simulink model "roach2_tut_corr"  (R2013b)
settings: Solver=VariableStepDiscrete  SolverMode=SingleTasking  StartTime=0.0  StopTime=100  RelTol=1e-3
undefined symbols (not defined in the file): add_latency, addr_width, Bit, bitfield, BitWidth, bram_latency, burst_size, casper_library_scopes, conv_latency, data_width, DelayLen, fan_latency, FFTSize, FFTStage, getfield, increment, led, Location, Lower, mult_latency, mux_latency, n_bits, n_bits_data, n_inputs, n_streams, n_taps, neg_latency, negate_latency, nsamples, pfb_size, pulse_len, reset_period, ROACH, ROACH2, snapshot, sx475t, sync_period, sync_period_bits, Upper, UseCounter, Width
libraries: xbsIndex_r4 x24444, casper_library_misc x73, xbsReplacements_r4 x34, casper_library_delays x14, xps_library x7
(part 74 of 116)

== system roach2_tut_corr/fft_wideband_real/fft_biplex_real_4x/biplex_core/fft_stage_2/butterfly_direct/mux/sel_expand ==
  bus_in : Inport
  reinterpret{1..16} (16 alike) : xbsIndex_r4/Reinterpret  force_arith_type=on  arith_type=Unsigned  force_bin_pt=on  bin_pt=0  block_type=reinterpret
  slice1 : xbsIndex_r4/Slice  nbits=1  boolean_output=off  mode=Upper Bit Location + Width  bit1=-15  base1=MSB of Input  bit0=0  base0=LSB of Input  dbl_ovrd=off  block_type=slice
  slice10 : xbsIndex_r4/Slice  nbits=1  boolean_output=off  mode=Upper Bit Location + Width  bit1=-6  base1=MSB of Input  bit0=0  base0=LSB of Input  dbl_ovrd=off  block_type=slice
  slice11 : xbsIndex_r4/Slice  nbits=1  boolean_output=off  mode=Upper Bit Location + Width  bit1=-5  base1=MSB of Input  bit0=0  base0=LSB of Input  dbl_ovrd=off  block_type=slice
  slice12 : xbsIndex_r4/Slice  nbits=1  boolean_output=off  mode=Upper Bit Location + Width  bit1=-4  base1=MSB of Input  bit0=0  base0=LSB of Input  dbl_ovrd=off  block_type=slice
  slice13 : xbsIndex_r4/Slice  nbits=1  boolean_output=off  mode=Upper Bit Location + Width  bit1=-3  base1=MSB of Input  bit0=0  base0=LSB of Input  dbl_ovrd=off  block_type=slice
  slice14 : xbsIndex_r4/Slice  nbits=1  boolean_output=off  mode=Upper Bit Location + Width  bit1=-2  base1=MSB of Input  bit0=0  base0=LSB of Input  dbl_ovrd=off  block_type=slice
  slice15 : xbsIndex_r4/Slice  nbits=1  boolean_output=off  mode=Upper Bit Location + Width  bit1=-1  base1=MSB of Input  bit0=0  base0=LSB of Input  dbl_ovrd=off  block_type=slice
  slice16 : xbsIndex_r4/Slice  nbits=1  boolean_output=off  mode=Upper Bit Location + Width  bit1=0  base1=MSB of Input  bit0=0  base0=LSB of Input  dbl_ovrd=off  block_type=slice
  slice2 : xbsIndex_r4/Slice  nbits=1  boolean_output=off  mode=Upper Bit Location + Width  bit1=-14  base1=MSB of Input  bit0=0  base0=LSB of Input  dbl_ovrd=off  block_type=slice
  slice3 : xbsIndex_r4/Slice  nbits=1  boolean_output=off  mode=Upper Bit Location + Width  bit1=-13  base1=MSB of Input  bit0=0  base0=LSB of Input  dbl_ovrd=off  block_type=slice
  slice4 : xbsIndex_r4/Slice  nbits=1  boolean_output=off  mode=Upper Bit Location + Width  bit1=-12  base1=MSB of Input  bit0=0  base0=LSB of Input  dbl_ovrd=off  block_type=slice
  slice5 : xbsIndex_r4/Slice  nbits=1  boolean_output=off  mode=Upper Bit Location + Width  bit1=-11  base1=MSB of Input  bit0=0  base0=LSB of Input  dbl_ovrd=off  block_type=slice
  slice6 : xbsIndex_r4/Slice  nbits=1  boolean_output=off  mode=Upper Bit Location + Width  bit1=-10  base1=MSB of Input  bit0=0  base0=LSB of Input  dbl_ovrd=off  block_type=slice
  slice7 : xbsIndex_r4/Slice  nbits=1  boolean_output=off  mode=Upper Bit Location + Width  bit1=-9  base1=MSB of Input  bit0=0  base0=LSB of Input  dbl_ovrd=off  block_type=slice
  slice8 : xbsIndex_r4/Slice  nbits=1  boolean_output=off  mode=Upper Bit Location + Width  bit1=-8  base1=MSB of Input  bit0=0  base0=LSB of Input  dbl_ovrd=off  block_type=slice
  slice9 : xbsIndex_r4/Slice  nbits=1  boolean_output=off  mode=Upper Bit Location + Width  bit1=-7  base1=MSB of Input  bit0=0  base0=LSB of Input  dbl_ovrd=off  block_type=slice
  msb_out16 : Outport
  out15 : Outport  Port=2
  out14 : Outport  Port=3
  out13 : Outport  Port=4
  out12 : Outport  Port=5
  out11 : Outport  Port=6
  out10 : Outport  Port=7
  out9 : Outport  Port=8
  out8 : Outport  Port=9
  out7 : Outport  Port=10
  out6 : Outport  Port=11
  out5 : Outport  Port=12
  out4 : Outport  Port=13
  out3 : Outport  Port=14
  out2 : Outport  Port=15
  lsb_out1 : Outport  Port=16
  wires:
  bus_in/1 -> slice16/1, slice15/1, slice14/1, slice13/1, slice12/1, slice11/1, slice10/1, slice9/1, slice8/1, slice7/1, slice6/1, slice5/1, slice4/1, slice3/1, slice2/1, slice1/1
  slice16/1 -> reinterpret16/1
  reinterpret16/1 -> msb_out16/1
  slice15/1 -> reinterpret15/1
  reinterpret15/1 -> out15/1
  slice14/1 -> reinterpret14/1
  reinterpret14/1 -> out14/1
  slice13/1 -> reinterpret13/1
  reinterpret13/1 -> out13/1
  slice12/1 -> reinterpret12/1
  reinterpret12/1 -> out12/1
  slice11/1 -> reinterpret11/1
  reinterpret11/1 -> out11/1
  slice10/1 -> reinterpret10/1
  reinterpret10/1 -> out10/1
  slice9/1 -> reinterpret9/1
  reinterpret9/1 -> out9/1
  slice8/1 -> reinterpret8/1
  reinterpret8/1 -> out8/1
  slice7/1 -> reinterpret7/1
  reinterpret7/1 -> out7/1
  slice6/1 -> reinterpret6/1
  reinterpret6/1 -> out6/1
  slice5/1 -> reinterpret5/1
  reinterpret5/1 -> out5/1
  slice4/1 -> reinterpret4/1
  reinterpret4/1 -> out4/1
  slice3/1 -> reinterpret3/1
  reinterpret3/1 -> out3/1
  slice2/1 -> reinterpret2/1
  reinterpret2/1 -> out2/1
  slice1/1 -> reinterpret1/1
  reinterpret1/1 -> lsb_out1/1

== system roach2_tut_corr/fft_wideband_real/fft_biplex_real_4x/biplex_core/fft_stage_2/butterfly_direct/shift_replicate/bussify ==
  in1 : Inport
  in2 : Inport  Port=2
  in3 : Inport  Port=3
  in4 : Inport  Port=4
  in5 : Inport  Port=5
  in6 : Inport  Port=6
  in7 : Inport  Port=7
  in8 : Inport  Port=8
  in9 : Inport  Port=9
  in10 : Inport  Port=10
  in11 : Inport  Port=11
  in12 : Inport  Port=12
  in13 : Inport  Port=13
  in14 : Inport  Port=14
  in15 : Inport  Port=15
  in16 : Inport  Port=16
  concatenate : xbsIndex_r4/Concat  num_inputs=16  dbl_ovrd=off  block_type=concat
  reinterpret{1..16} (16 alike) : xbsIndex_r4/Reinterpret  force_arith_type=on  arith_type=Unsigned  force_bin_pt=on  bin_pt=0  block_type=reinterpret
  bus_out : Outport
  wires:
  concatenate/1 -> bus_out/1
  in1/1 -> reinterpret1/1
  reinterpret1/1 -> concatenate/1
  in2/1 -> reinterpret2/1
  reinterpret2/1 -> concatenate/2
  in3/1 -> reinterpret3/1
  reinterpret3/1 -> concatenate/3
  in4/1 -> reinterpret4/1
  reinterpret4/1 -> concatenate/4
  in5/1 -> reinterpret5/1
  reinterpret5/1 -> concatenate/5
  in6/1 -> reinterpret6/1
  reinterpret6/1 -> concatenate/6
  in7/1 -> reinterpret7/1
  reinterpret7/1 -> concatenate/7
  in8/1 -> reinterpret8/1
  reinterpret8/1 -> concatenate/8
  in9/1 -> reinterpret9/1
  reinterpret9/1 -> concatenate/9
  in10/1 -> reinterpret10/1
  reinterpret10/1 -> concatenate/10
  in11/1 -> reinterpret11/1
  reinterpret11/1 -> concatenate/11
  in12/1 -> reinterpret12/1
  reinterpret12/1 -> concatenate/12
  in13/1 -> reinterpret13/1
  reinterpret13/1 -> concatenate/13
  in14/1 -> reinterpret14/1
  reinterpret14/1 -> concatenate/14
  in15/1 -> reinterpret15/1
  reinterpret15/1 -> concatenate/15
  in16/1 -> reinterpret16/1
  reinterpret16/1 -> concatenate/16

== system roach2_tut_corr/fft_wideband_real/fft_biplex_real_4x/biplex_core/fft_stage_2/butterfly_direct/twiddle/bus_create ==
  in1 : Inport
  in2 : Inport  Port=2
  concatenate : xbsIndex_r4/Concat  num_inputs=2  dbl_ovrd=off  block_type=concat
  reinterpret1 : xbsIndex_r4/Reinterpret  force_arith_type=on  arith_type=Unsigned  force_bin_pt=on  bin_pt=0  block_type=reinterpret
  reinterpret2 : xbsIndex_r4/Reinterpret  force_arith_type=on  arith_type=Unsigned  force_bin_pt=on  bin_pt=0  block_type=reinterpret
  bus_out : Outport
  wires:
  concatenate/1 -> bus_out/1
  in1/1 -> reinterpret1/1
  reinterpret1/1 -> concatenate/1
  in2/1 -> reinterpret2/1
  reinterpret2/1 -> concatenate/2

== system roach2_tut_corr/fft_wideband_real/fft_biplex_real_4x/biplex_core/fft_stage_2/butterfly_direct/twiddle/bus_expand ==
  bus_in : Inport
  reinterpret1 : xbsIndex_r4/Reinterpret  force_arith_type=on  arith_type=Unsigned  force_bin_pt=on  bin_pt=0  block_type=reinterpret
  reinterpret2 : xbsIndex_r4/Reinterpret  force_arith_type=on  arith_type=Unsigned  force_bin_pt=on  bin_pt=0  block_type=reinterpret
  slice1 : xbsIndex_r4/Slice  nbits=72  boolean_output=off  mode=Upper Bit Location + Width  bit1=-72  base1=MSB of Input  bit0=0  base0=LSB of Input  dbl_ovrd=off  block_type=slice
  slice2 : xbsIndex_r4/Slice  nbits=72  boolean_output=off  mode=Upper Bit Location + Width  bit1=0  base1=MSB of Input  bit0=0  base0=LSB of Input  dbl_ovrd=off  block_type=slice
  msb_out2 : Outport
  lsb_out1 : Outport  Port=2
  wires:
  bus_in/1 -> slice2/1, slice1/1
  slice2/1 -> reinterpret2/1
  reinterpret2/1 -> msb_out2/1
  slice1/1 -> reinterpret1/1
  reinterpret1/1 -> lsb_out1/1

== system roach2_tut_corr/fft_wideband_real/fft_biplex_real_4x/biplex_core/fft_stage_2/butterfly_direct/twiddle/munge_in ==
  din : Inport
  join : Subsystem  AncestorBlock=casper_library_flow_control/bus_create
  reinterpret : xbsIndex_r4/Reinterpret  force_arith_type=on  arith_type=Unsigned  force_bin_pt=on  bin_pt=0  block_type=reinterpret
  reinterpret_out : xbsIndex_r4/Reinterpret  force_arith_type=on  arith_type=Unsigned  force_bin_pt=on  bin_pt=0  block_type=reinterpret
  split : Subsystem  AncestorBlock=casper_library_flow_control/bus_expand
  dout : Outport
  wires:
  reinterpret_out/1 -> dout/1
  din/1 -> reinterpret/1
  reinterpret/1 -> split/1(bus_in)
  join/1(bus_out) -> reinterpret_out/1
  split/1(msb_out8) -> join/1(in1)
  split/3(out6) -> join/2(in2)
  split/5(out4) -> join/3(in3)
  split/7(out2) -> join/4(in4)
  split/2(out7) -> join/5(in5)
  split/4(out5) -> join/6(in6)
  split/6(out3) -> join/7(in7)
  split/8(lsb_out1) -> join/8(in8)

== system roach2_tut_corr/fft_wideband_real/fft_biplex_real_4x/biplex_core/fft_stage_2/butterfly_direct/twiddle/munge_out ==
  din : Inport
  join : Subsystem  AncestorBlock=casper_library_flow_control/bus_create
  reinterpret : xbsIndex_r4/Reinterpret  force_arith_type=on  arith_type=Unsigned  force_bin_pt=on  bin_pt=0  block_type=reinterpret
  reinterpret_out : xbsIndex_r4/Reinterpret  force_arith_type=on  arith_type=Unsigned  force_bin_pt=on  bin_pt=0  block_type=reinterpret
  split : Subsystem  AncestorBlock=casper_library_flow_control/bus_expand
  dout : Outport
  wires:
  reinterpret_out/1 -> dout/1
  din/1 -> reinterpret/1
  reinterpret/1 -> split/1(bus_in)
  join/1(bus_out) -> reinterpret_out/1
  split/1(msb_out8) -> join/1(in1)
  split/5(out4) -> join/2(in2)
  split/2(out7) -> join/3(in3)
  split/6(out3) -> join/4(in4)
  split/3(out6) -> join/5(in5)
  split/7(out2) -> join/6(in6)
  split/4(out5) -> join/7(in7)
  split/8(lsb_out1) -> join/8(in8)

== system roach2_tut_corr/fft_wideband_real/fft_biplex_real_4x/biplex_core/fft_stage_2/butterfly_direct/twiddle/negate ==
  din : Inport
  bussify : Subsystem  AncestorBlock=casper_library_flow_control/bus_create
  debus : Subsystem  AncestorBlock=casper_library_flow_control/bus_expand
  neg{1..4} (4 alike) : xbsIndex_r4/Negate  precision=User Defined  arith_type="Signed  (2's comp)"  n_bits=18  bin_pt=17  quantization=Truncate  overflow=Saturate  en=off  latency=latency  dbl_ovrd=off  block_type=negate
  dout : Outport
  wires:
  din/1 -> debus/1(bus_in)
  debus/1(msb_out4) -> neg1/1
  debus/2(out3) -> neg2/1
  debus/3(out2) -> neg3/1
  debus/4(lsb_out1) -> neg4/1
  neg1/1 -> bussify/1(in1)
  neg2/1 -> bussify/2(in2)
  neg3/1 -> bussify/3(in3)
  neg4/1 -> bussify/4(in4)
  bussify/1(bus_out) -> dout/1

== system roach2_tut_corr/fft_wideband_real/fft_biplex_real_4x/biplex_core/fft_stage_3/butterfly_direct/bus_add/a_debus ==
  bus_in : Inport
  reinterpret{1..8} (8 alike) : xbsIndex_r4/Reinterpret  force_arith_type=on  arith_type="Signed  (2's comp)"  force_bin_pt=on  bin_pt=17  block_type=reinterpret
  slice1 : xbsIndex_r4/Slice  nbits=18  boolean_output=off  mode=Upper Bit Location + Width  bit1=-126  base1=MSB of Input  bit0=0  base0=LSB of Input  dbl_ovrd=off  block_type=slice
  slice2 : xbsIndex_r4/Slice  nbits=18  boolean_output=off  mode=Upper Bit Location + Width  bit1=-108  base1=MSB of Input  bit0=0  base0=LSB of Input  dbl_ovrd=off  block_type=slice
  slice3 : xbsIndex_r4/Slice  nbits=18  boolean_output=off  mode=Upper Bit Location + Width  bit1=-90  base1=MSB of Input  bit0=0  base0=LSB of Input  dbl_ovrd=off  block_type=slice
  slice4 : xbsIndex_r4/Slice  nbits=18  boolean_output=off  mode=Upper Bit Location + Width  bit1=-72  base1=MSB of Input  bit0=0  base0=LSB of Input  dbl_ovrd=off  block_type=slice
  slice5 : xbsIndex_r4/Slice  nbits=18  boolean_output=off  mode=Upper Bit Location + Width  bit1=-54  base1=MSB of Input  bit0=0  base0=LSB of Input  dbl_ovrd=off  block_type=slice
  slice6 : xbsIndex_r4/Slice  nbits=18  boolean_output=off  mode=Upper Bit Location + Width  bit1=-36  base1=MSB of Input  bit0=0  base0=LSB of Input  dbl_ovrd=off  block_type=slice
  slice7 : xbsIndex_r4/Slice  nbits=18  boolean_output=off  mode=Upper Bit Location + Width  bit1=-18  base1=MSB of Input  bit0=0  base0=LSB of Input  dbl_ovrd=off  block_type=slice
  slice8 : xbsIndex_r4/Slice  nbits=18  boolean_output=off  mode=Upper Bit Location + Width  bit1=0  base1=MSB of Input  bit0=0  base0=LSB of Input  dbl_ovrd=off  block_type=slice
  msb_out8 : Outport
  out7 : Outport  Port=2
  out6 : Outport  Port=3
  out5 : Outport  Port=4
  out4 : Outport  Port=5
  out3 : Outport  Port=6
  out2 : Outport  Port=7
  lsb_out1 : Outport  Port=8
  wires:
  bus_in/1 -> slice8/1, slice7/1, slice6/1, slice5/1, slice4/1, slice3/1, slice2/1, slice1/1
  slice8/1 -> reinterpret8/1
  reinterpret8/1 -> msb_out8/1
  slice7/1 -> reinterpret7/1
  reinterpret7/1 -> out7/1
  slice6/1 -> reinterpret6/1
  reinterpret6/1 -> out6/1
  slice5/1 -> reinterpret5/1
  reinterpret5/1 -> out5/1
  slice4/1 -> reinterpret4/1
  reinterpret4/1 -> out4/1
  slice3/1 -> reinterpret3/1
  reinterpret3/1 -> out3/1
  slice2/1 -> reinterpret2/1
  reinterpret2/1 -> out2/1
  slice1/1 -> reinterpret1/1
  reinterpret1/1 -> lsb_out1/1

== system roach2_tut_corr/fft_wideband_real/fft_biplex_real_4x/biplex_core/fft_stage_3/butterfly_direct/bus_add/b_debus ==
  bus_in : Inport
  reinterpret{1..8} (8 alike) : xbsIndex_r4/Reinterpret  force_arith_type=on  arith_type="Signed  (2's comp)"  force_bin_pt=on  bin_pt=17  block_type=reinterpret
  slice1 : xbsIndex_r4/Slice  nbits=19  boolean_output=off  mode=Upper Bit Location + Width  bit1=-133  base1=MSB of Input  bit0=0  base0=LSB of Input  dbl_ovrd=off  block_type=slice
  slice2 : xbsIndex_r4/Slice  nbits=19  boolean_output=off  mode=Upper Bit Location + Width  bit1=-114  base1=MSB of Input  bit0=0  base0=LSB of Input  dbl_ovrd=off  block_type=slice
  slice3 : xbsIndex_r4/Slice  nbits=19  boolean_output=off  mode=Upper Bit Location + Width  bit1=-95  base1=MSB of Input  bit0=0  base0=LSB of Input  dbl_ovrd=off  block_type=slice
  slice4 : xbsIndex_r4/Slice  nbits=19  boolean_output=off  mode=Upper Bit Location + Width  bit1=-76  base1=MSB of Input  bit0=0  base0=LSB of Input  dbl_ovrd=off  block_type=slice
  slice5 : xbsIndex_r4/Slice  nbits=19  boolean_output=off  mode=Upper Bit Location + Width  bit1=-57  base1=MSB of Input  bit0=0  base0=LSB of Input  dbl_ovrd=off  block_type=slice
  slice6 : xbsIndex_r4/Slice  nbits=19  boolean_output=off  mode=Upper Bit Location + Width  bit1=-38  base1=MSB of Input  bit0=0  base0=LSB of Input  dbl_ovrd=off  block_type=slice
  slice7 : xbsIndex_r4/Slice  nbits=19  boolean_output=off  mode=Upper Bit Location + Width  bit1=-19  base1=MSB of Input  bit0=0  base0=LSB of Input  dbl_ovrd=off  block_type=slice
  slice8 : xbsIndex_r4/Slice  nbits=19  boolean_output=off  mode=Upper Bit Location + Width  bit1=0  base1=MSB of Input  bit0=0  base0=LSB of Input  dbl_ovrd=off  block_type=slice
  msb_out8 : Outport
  out7 : Outport  Port=2
  out6 : Outport  Port=3
  out5 : Outport  Port=4
  out4 : Outport  Port=5
  out3 : Outport  Port=6
  out2 : Outport  Port=7
  lsb_out1 : Outport  Port=8
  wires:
  bus_in/1 -> slice8/1, slice7/1, slice6/1, slice5/1, slice4/1, slice3/1, slice2/1, slice1/1
  slice8/1 -> reinterpret8/1
  reinterpret8/1 -> msb_out8/1
  slice7/1 -> reinterpret7/1
  reinterpret7/1 -> out7/1
  slice6/1 -> reinterpret6/1
  reinterpret6/1 -> out6/1
  slice5/1 -> reinterpret5/1
  reinterpret5/1 -> out5/1
  slice4/1 -> reinterpret4/1
  reinterpret4/1 -> out4/1
  slice3/1 -> reinterpret3/1
  reinterpret3/1 -> out3/1
  slice2/1 -> reinterpret2/1
  reinterpret2/1 -> out2/1
  slice1/1 -> reinterpret1/1
  reinterpret1/1 -> lsb_out1/1

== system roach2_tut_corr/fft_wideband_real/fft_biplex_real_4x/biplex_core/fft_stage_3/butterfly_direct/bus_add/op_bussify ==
  in1 : Inport
  in2 : Inport  Port=2
  in3 : Inport  Port=3
  in4 : Inport  Port=4
  in5 : Inport  Port=5
  in6 : Inport  Port=6
  in7 : Inport  Port=7
  in8 : Inport  Port=8
  concatenate : xbsIndex_r4/Concat  num_inputs=8  dbl_ovrd=off  block_type=concat
  reinterpret{1..8} (8 alike) : xbsIndex_r4/Reinterpret  force_arith_type=on  arith_type=Unsigned  force_bin_pt=on  bin_pt=0  block_type=reinterpret
  bus_out : Outport
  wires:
  concatenate/1 -> bus_out/1
  in1/1 -> reinterpret1/1
  reinterpret1/1 -> concatenate/1
  in2/1 -> reinterpret2/1
  reinterpret2/1 -> concatenate/2
  in3/1 -> reinterpret3/1
  reinterpret3/1 -> concatenate/3
  in4/1 -> reinterpret4/1
  reinterpret4/1 -> concatenate/4
  in5/1 -> reinterpret5/1
  reinterpret5/1 -> concatenate/5
  in6/1 -> reinterpret6/1
  reinterpret6/1 -> concatenate/6
  in7/1 -> reinterpret7/1
  reinterpret7/1 -> concatenate/7
  in8/1 -> reinterpret8/1
  reinterpret8/1 -> concatenate/8

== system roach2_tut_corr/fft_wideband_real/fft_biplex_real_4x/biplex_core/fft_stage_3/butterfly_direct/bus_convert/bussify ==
  in1 : Inport
  in2 : Inport  Port=2
  in3 : Inport  Port=3
  in4 : Inport  Port=4
  in5 : Inport  Port=5
  in6 : Inport  Port=6
  in7 : Inport  Port=7
  in8 : Inport  Port=8
  in9 : Inport  Port=9
  in10 : Inport  Port=10
  in11 : Inport  Port=11
  in12 : Inport  Port=12
  in13 : Inport  Port=13
  in14 : Inport  Port=14
  in15 : Inport  Port=15
  in16 : Inport  Port=16
  concatenate : xbsIndex_r4/Concat  num_inputs=16  dbl_ovrd=off  block_type=concat
  reinterpret{1..16} (16 alike) : xbsIndex_r4/Reinterpret  force_arith_type=on  arith_type=Unsigned  force_bin_pt=on  bin_pt=0  block_type=reinterpret
  bus_out : Outport
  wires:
  concatenate/1 -> bus_out/1
  in1/1 -> reinterpret1/1
  reinterpret1/1 -> concatenate/1
  in2/1 -> reinterpret2/1
  reinterpret2/1 -> concatenate/2
  in3/1 -> reinterpret3/1
  reinterpret3/1 -> concatenate/3
  in4/1 -> reinterpret4/1
  reinterpret4/1 -> concatenate/4
  in5/1 -> reinterpret5/1
  reinterpret5/1 -> concatenate/5
  in6/1 -> reinterpret6/1
  reinterpret6/1 -> concatenate/6
  in7/1 -> reinterpret7/1
  reinterpret7/1 -> concatenate/7
  in8/1 -> reinterpret8/1
  reinterpret8/1 -> concatenate/8
  in9/1 -> reinterpret9/1
  reinterpret9/1 -> concatenate/9
  in10/1 -> reinterpret10/1
  reinterpret10/1 -> concatenate/10
  in11/1 -> reinterpret11/1
  reinterpret11/1 -> concatenate/11
  in12/1 -> reinterpret12/1
  reinterpret12/1 -> concatenate/12
  in13/1 -> reinterpret13/1
  reinterpret13/1 -> concatenate/13
  in14/1 -> reinterpret14/1
  reinterpret14/1 -> concatenate/14
  in15/1 -> reinterpret15/1
  reinterpret15/1 -> concatenate/15
  in16/1 -> reinterpret16/1
  reinterpret16/1 -> concatenate/16

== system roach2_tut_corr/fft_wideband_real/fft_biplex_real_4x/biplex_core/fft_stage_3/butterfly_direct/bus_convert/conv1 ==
  din : Inport
  all_0s : xbsIndex_r4/Logical  logical_function=NAND  inputs=3  en=off  latency=1  precision=Full  arith_type=Unsigned  n_bits=16  bin_pt=0  align_bp=on  dbl_ovrd=off  block_type=logical
  all_1s : xbsIndex_r4/Logical  logical_function=NAND  inputs=3  en=off  latency=1  precision=Full  arith_type=Unsigned  n_bits=16  bin_pt=0  align_bp=on  dbl_ovrd=off  block_type=logical
  and : xbsIndex_r4/Logical  logical_function=AND  inputs=2  en=off  latency=0  precision=Full  arith_type=Unsigned  n_bits=16  bin_pt=0  align_bp=on  dbl_ovrd=off  block_type=logical
  convert : Subsystem  AncestorBlock=casper_library_misc/convert
  invert1 : xbsIndex_r4/Inverter  en=off  latency=0  dbl_ovrd=off  block_type=inv
  invert2 : xbsIndex_r4/Inverter  en=off  latency=0  dbl_ovrd=off  block_type=inv
  invert3 : xbsIndex_r4/Inverter  en=off  latency=0  dbl_ovrd=off  block_type=inv
  slice1 : xbsIndex_r4/Slice  nbits=1  boolean_output=on  mode=Upper Bit Location + Width  bit1=0  base1=MSB of Input  bit0=0  base0=LSB of Input  dbl_ovrd=off  block_type=slice
  slice2 : xbsIndex_r4/Slice  nbits=1  boolean_output=on  mode=Upper Bit Location + Width  bit1=-1  base1=MSB of Input  bit0=0  base0=LSB of Input  dbl_ovrd=off  block_type=slice
  slice3 : xbsIndex_r4/Slice  nbits=1  boolean_output=on  mode=Upper Bit Location + Width  bit1=-2  base1=MSB of Input  bit0=0  base0=LSB of Input  dbl_ovrd=off  block_type=slice
  dout : Outport
  of : Outport  Port=2
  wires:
  din/1 -> convert/1(in), slice1/1, slice2/1, slice3/1
  convert/1(out) -> dout/1
  slice1/1 -> all_1s/1, invert1/1
  invert1/1 -> all_0s/1
  slice2/1 -> all_1s/2, invert2/1
  invert2/1 -> all_0s/2
  slice3/1 -> all_1s/3, invert3/1
  invert3/1 -> all_0s/3
  all_0s/1 -> and/1
  all_1s/1 -> and/2
  and/1 -> of/1

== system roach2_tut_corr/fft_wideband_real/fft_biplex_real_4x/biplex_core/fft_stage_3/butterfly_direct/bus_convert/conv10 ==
  din : Inport
  all_0s : xbsIndex_r4/Logical  logical_function=NAND  inputs=3  en=off  latency=1  precision=Full  arith_type=Unsigned  n_bits=16  bin_pt=0  align_bp=on  dbl_ovrd=off  block_type=logical
  all_1s : xbsIndex_r4/Logical  logical_function=NAND  inputs=3  en=off  latency=1  precision=Full  arith_type=Unsigned  n_bits=16  bin_pt=0  align_bp=on  dbl_ovrd=off  block_type=logical
  and : xbsIndex_r4/Logical  logical_function=AND  inputs=2  en=off  latency=0  precision=Full  arith_type=Unsigned  n_bits=16  bin_pt=0  align_bp=on  dbl_ovrd=off  block_type=logical
  convert : Subsystem  AncestorBlock=casper_library_misc/convert
  invert1 : xbsIndex_r4/Inverter  en=off  latency=0  dbl_ovrd=off  block_type=inv
  invert2 : xbsIndex_r4/Inverter  en=off  latency=0  dbl_ovrd=off  block_type=inv
  invert3 : xbsIndex_r4/Inverter  en=off  latency=0  dbl_ovrd=off  block_type=inv
  slice1 : xbsIndex_r4/Slice  nbits=1  boolean_output=on  mode=Upper Bit Location + Width  bit1=0  base1=MSB of Input  bit0=0  base0=LSB of Input  dbl_ovrd=off  block_type=slice
  slice2 : xbsIndex_r4/Slice  nbits=1  boolean_output=on  mode=Upper Bit Location + Width  bit1=-1  base1=MSB of Input  bit0=0  base0=LSB of Input  dbl_ovrd=off  block_type=slice
  slice3 : xbsIndex_r4/Slice  nbits=1  boolean_output=on  mode=Upper Bit Location + Width  bit1=-2  base1=MSB of Input  bit0=0  base0=LSB of Input  dbl_ovrd=off  block_type=slice
  dout : Outport
  of : Outport  Port=2
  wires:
  din/1 -> convert/1(in), slice1/1, slice2/1, slice3/1
  convert/1(out) -> dout/1
  slice1/1 -> all_1s/1, invert1/1
  invert1/1 -> all_0s/1
  slice2/1 -> all_1s/2, invert2/1
  invert2/1 -> all_0s/2
  slice3/1 -> all_1s/3, invert3/1
  invert3/1 -> all_0s/3
  all_0s/1 -> and/1
  all_1s/1 -> and/2
  and/1 -> of/1

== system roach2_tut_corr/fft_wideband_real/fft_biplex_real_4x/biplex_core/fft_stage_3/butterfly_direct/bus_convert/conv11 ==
  din : Inport
  all_0s : xbsIndex_r4/Logical  logical_function=NAND  inputs=3  en=off  latency=1  precision=Full  arith_type=Unsigned  n_bits=16  bin_pt=0  align_bp=on  dbl_ovrd=off  block_type=logical
  all_1s : xbsIndex_r4/Logical  logical_function=NAND  inputs=3  en=off  latency=1  precision=Full  arith_type=Unsigned  n_bits=16  bin_pt=0  align_bp=on  dbl_ovrd=off  block_type=logical
  and : xbsIndex_r4/Logical  logical_function=AND  inputs=2  en=off  latency=0  precision=Full  arith_type=Unsigned  n_bits=16  bin_pt=0  align_bp=on  dbl_ovrd=off  block_type=logical
  convert : Subsystem  AncestorBlock=casper_library_misc/convert
  invert1 : xbsIndex_r4/Inverter  en=off  latency=0  dbl_ovrd=off  block_type=inv
  invert2 : xbsIndex_r4/Inverter  en=off  latency=0  dbl_ovrd=off  block_type=inv
  invert3 : xbsIndex_r4/Inverter  en=off  latency=0  dbl_ovrd=off  block_type=inv
  slice1 : xbsIndex_r4/Slice  nbits=1  boolean_output=on  mode=Upper Bit Location + Width  bit1=0  base1=MSB of Input  bit0=0  base0=LSB of Input  dbl_ovrd=off  block_type=slice
  slice2 : xbsIndex_r4/Slice  nbits=1  boolean_output=on  mode=Upper Bit Location + Width  bit1=-1  base1=MSB of Input  bit0=0  base0=LSB of Input  dbl_ovrd=off  block_type=slice
  slice3 : xbsIndex_r4/Slice  nbits=1  boolean_output=on  mode=Upper Bit Location + Width  bit1=-2  base1=MSB of Input  bit0=0  base0=LSB of Input  dbl_ovrd=off  block_type=slice
  dout : Outport
  of : Outport  Port=2
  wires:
  din/1 -> convert/1(in), slice1/1, slice2/1, slice3/1
  convert/1(out) -> dout/1
  slice1/1 -> all_1s/1, invert1/1
  invert1/1 -> all_0s/1
  slice2/1 -> all_1s/2, invert2/1
  invert2/1 -> all_0s/2
  slice3/1 -> all_1s/3, invert3/1
  invert3/1 -> all_0s/3
  all_0s/1 -> and/1
  all_1s/1 -> and/2
  and/1 -> of/1

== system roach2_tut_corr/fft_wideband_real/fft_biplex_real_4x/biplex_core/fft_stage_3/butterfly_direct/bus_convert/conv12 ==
  din : Inport
  all_0s : xbsIndex_r4/Logical  logical_function=NAND  inputs=3  en=off  latency=1  precision=Full  arith_type=Unsigned  n_bits=16  bin_pt=0  align_bp=on  dbl_ovrd=off  block_type=logical
  all_1s : xbsIndex_r4/Logical  logical_function=NAND  inputs=3  en=off  latency=1  precision=Full  arith_type=Unsigned  n_bits=16  bin_pt=0  align_bp=on  dbl_ovrd=off  block_type=logical
  and : xbsIndex_r4/Logical  logical_function=AND  inputs=2  en=off  latency=0  precision=Full  arith_type=Unsigned  n_bits=16  bin_pt=0  align_bp=on  dbl_ovrd=off  block_type=logical
  convert : Subsystem  AncestorBlock=casper_library_misc/convert
  invert1 : xbsIndex_r4/Inverter  en=off  latency=0  dbl_ovrd=off  block_type=inv
  invert2 : xbsIndex_r4/Inverter  en=off  latency=0  dbl_ovrd=off  block_type=inv
  invert3 : xbsIndex_r4/Inverter  en=off  latency=0  dbl_ovrd=off  block_type=inv
  slice1 : xbsIndex_r4/Slice  nbits=1  boolean_output=on  mode=Upper Bit Location + Width  bit1=0  base1=MSB of Input  bit0=0  base0=LSB of Input  dbl_ovrd=off  block_type=slice
  slice2 : xbsIndex_r4/Slice  nbits=1  boolean_output=on  mode=Upper Bit Location + Width  bit1=-1  base1=MSB of Input  bit0=0  base0=LSB of Input  dbl_ovrd=off  block_type=slice
  slice3 : xbsIndex_r4/Slice  nbits=1  boolean_output=on  mode=Upper Bit Location + Width  bit1=-2  base1=MSB of Input  bit0=0  base0=LSB of Input  dbl_ovrd=off  block_type=slice
  dout : Outport
  of : Outport  Port=2
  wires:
  din/1 -> convert/1(in), slice1/1, slice2/1, slice3/1
  convert/1(out) -> dout/1
  slice1/1 -> all_1s/1, invert1/1
  invert1/1 -> all_0s/1
  slice2/1 -> all_1s/2, invert2/1
  invert2/1 -> all_0s/2
  slice3/1 -> all_1s/3, invert3/1
  invert3/1 -> all_0s/3
  all_0s/1 -> and/1
  all_1s/1 -> and/2
  and/1 -> of/1

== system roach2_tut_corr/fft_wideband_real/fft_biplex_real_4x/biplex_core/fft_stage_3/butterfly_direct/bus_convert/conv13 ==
  din : Inport
  all_0s : xbsIndex_r4/Logical  logical_function=NAND  inputs=3  en=off  latency=1  precision=Full  arith_type=Unsigned  n_bits=16  bin_pt=0  align_bp=on  dbl_ovrd=off  block_type=logical
  all_1s : xbsIndex_r4/Logical  logical_function=NAND  inputs=3  en=off  latency=1  precision=Full  arith_type=Unsigned  n_bits=16  bin_pt=0  align_bp=on  dbl_ovrd=off  block_type=logical
  and : xbsIndex_r4/Logical  logical_function=AND  inputs=2  en=off  latency=0  precision=Full  arith_type=Unsigned  n_bits=16  bin_pt=0  align_bp=on  dbl_ovrd=off  block_type=logical
  convert : Subsystem  AncestorBlock=casper_library_misc/convert
  invert1 : xbsIndex_r4/Inverter  en=off  latency=0  dbl_ovrd=off  block_type=inv
  invert2 : xbsIndex_r4/Inverter  en=off  latency=0  dbl_ovrd=off  block_type=inv
  invert3 : xbsIndex_r4/Inverter  en=off  latency=0  dbl_ovrd=off  block_type=inv
  slice1 : xbsIndex_r4/Slice  nbits=1  boolean_output=on  mode=Upper Bit Location + Width  bit1=0  base1=MSB of Input  bit0=0  base0=LSB of Input  dbl_ovrd=off  block_type=slice
  slice2 : xbsIndex_r4/Slice  nbits=1  boolean_output=on  mode=Upper Bit Location + Width  bit1=-1  base1=MSB of Input  bit0=0  base0=LSB of Input  dbl_ovrd=off  block_type=slice
  slice3 : xbsIndex_r4/Slice  nbits=1  boolean_output=on  mode=Upper Bit Location + Width  bit1=-2  base1=MSB of Input  bit0=0  base0=LSB of Input  dbl_ovrd=off  block_type=slice
  dout : Outport
  of : Outport  Port=2
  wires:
  din/1 -> convert/1(in), slice1/1, slice2/1, slice3/1
  convert/1(out) -> dout/1
  slice1/1 -> all_1s/1, invert1/1
  invert1/1 -> all_0s/1
  slice2/1 -> all_1s/2, invert2/1
  invert2/1 -> all_0s/2
  slice3/1 -> all_1s/3, invert3/1
  invert3/1 -> all_0s/3
  all_0s/1 -> and/1
  all_1s/1 -> and/2
  and/1 -> of/1

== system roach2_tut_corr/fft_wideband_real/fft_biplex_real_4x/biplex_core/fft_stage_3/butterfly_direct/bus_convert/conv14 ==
  din : Inport
  all_0s : xbsIndex_r4/Logical  logical_function=NAND  inputs=3  en=off  latency=1  precision=Full  arith_type=Unsigned  n_bits=16  bin_pt=0  align_bp=on  dbl_ovrd=off  block_type=logical
  all_1s : xbsIndex_r4/Logical  logical_function=NAND  inputs=3  en=off  latency=1  precision=Full  arith_type=Unsigned  n_bits=16  bin_pt=0  align_bp=on  dbl_ovrd=off  block_type=logical
  and : xbsIndex_r4/Logical  logical_function=AND  inputs=2  en=off  latency=0  precision=Full  arith_type=Unsigned  n_bits=16  bin_pt=0  align_bp=on  dbl_ovrd=off  block_type=logical
  convert : Subsystem  AncestorBlock=casper_library_misc/convert
  invert1 : xbsIndex_r4/Inverter  en=off  latency=0  dbl_ovrd=off  block_type=inv
  invert2 : xbsIndex_r4/Inverter  en=off  latency=0  dbl_ovrd=off  block_type=inv
  invert3 : xbsIndex_r4/Inverter  en=off  latency=0  dbl_ovrd=off  block_type=inv
  slice1 : xbsIndex_r4/Slice  nbits=1  boolean_output=on  mode=Upper Bit Location + Width  bit1=0  base1=MSB of Input  bit0=0  base0=LSB of Input  dbl_ovrd=off  block_type=slice
  slice2 : xbsIndex_r4/Slice  nbits=1  boolean_output=on  mode=Upper Bit Location + Width  bit1=-1  base1=MSB of Input  bit0=0  base0=LSB of Input  dbl_ovrd=off  block_type=slice
  slice3 : xbsIndex_r4/Slice  nbits=1  boolean_output=on  mode=Upper Bit Location + Width  bit1=-2  base1=MSB of Input  bit0=0  base0=LSB of Input  dbl_ovrd=off  block_type=slice
  dout : Outport
  of : Outport  Port=2
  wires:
  din/1 -> convert/1(in), slice1/1, slice2/1, slice3/1
  convert/1(out) -> dout/1
  slice1/1 -> all_1s/1, invert1/1
  invert1/1 -> all_0s/1
  slice2/1 -> all_1s/2, invert2/1
  invert2/1 -> all_0s/2
  slice3/1 -> all_1s/3, invert3/1
  invert3/1 -> all_0s/3
  all_0s/1 -> and/1
  all_1s/1 -> and/2
  and/1 -> of/1

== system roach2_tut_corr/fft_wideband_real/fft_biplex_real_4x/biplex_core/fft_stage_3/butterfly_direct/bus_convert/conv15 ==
  din : Inport
  all_0s : xbsIndex_r4/Logical  logical_function=NAND  inputs=3  en=off  latency=1  precision=Full  arith_type=Unsigned  n_bits=16  bin_pt=0  align_bp=on  dbl_ovrd=off  block_type=logical
  all_1s : xbsIndex_r4/Logical  logical_function=NAND  inputs=3  en=off  latency=1  precision=Full  arith_type=Unsigned  n_bits=16  bin_pt=0  align_bp=on  dbl_ovrd=off  block_type=logical
  and : xbsIndex_r4/Logical  logical_function=AND  inputs=2  en=off  latency=0  precision=Full  arith_type=Unsigned  n_bits=16  bin_pt=0  align_bp=on  dbl_ovrd=off  block_type=logical
  convert : Subsystem  AncestorBlock=casper_library_misc/convert
  invert1 : xbsIndex_r4/Inverter  en=off  latency=0  dbl_ovrd=off  block_type=inv
  invert2 : xbsIndex_r4/Inverter  en=off  latency=0  dbl_ovrd=off  block_type=inv
  invert3 : xbsIndex_r4/Inverter  en=off  latency=0  dbl_ovrd=off  block_type=inv
  slice1 : xbsIndex_r4/Slice  nbits=1  boolean_output=on  mode=Upper Bit Location + Width  bit1=0  base1=MSB of Input  bit0=0  base0=LSB of Input  dbl_ovrd=off  block_type=slice
  slice2 : xbsIndex_r4/Slice  nbits=1  boolean_output=on  mode=Upper Bit Location + Width  bit1=-1  base1=MSB of Input  bit0=0  base0=LSB of Input  dbl_ovrd=off  block_type=slice
  slice3 : xbsIndex_r4/Slice  nbits=1  boolean_output=on  mode=Upper Bit Location + Width  bit1=-2  base1=MSB of Input  bit0=0  base0=LSB of Input  dbl_ovrd=off  block_type=slice
  dout : Outport
  of : Outport  Port=2
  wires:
  din/1 -> convert/1(in), slice1/1, slice2/1, slice3/1
  convert/1(out) -> dout/1
  slice1/1 -> all_1s/1, invert1/1
  invert1/1 -> all_0s/1
  slice2/1 -> all_1s/2, invert2/1
  invert2/1 -> all_0s/2
  slice3/1 -> all_1s/3, invert3/1
  invert3/1 -> all_0s/3
  all_0s/1 -> and/1
  all_1s/1 -> and/2
  and/1 -> of/1

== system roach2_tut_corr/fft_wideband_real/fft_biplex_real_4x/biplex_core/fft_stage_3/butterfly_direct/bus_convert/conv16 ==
  din : Inport
  all_0s : xbsIndex_r4/Logical  logical_function=NAND  inputs=3  en=off  latency=1  precision=Full  arith_type=Unsigned  n_bits=16  bin_pt=0  align_bp=on  dbl_ovrd=off  block_type=logical
  all_1s : xbsIndex_r4/Logical  logical_function=NAND  inputs=3  en=off  latency=1  precision=Full  arith_type=Unsigned  n_bits=16  bin_pt=0  align_bp=on  dbl_ovrd=off  block_type=logical
  and : xbsIndex_r4/Logical  logical_function=AND  inputs=2  en=off  latency=0  precision=Full  arith_type=Unsigned  n_bits=16  bin_pt=0  align_bp=on  dbl_ovrd=off  block_type=logical
  convert : Subsystem  AncestorBlock=casper_library_misc/convert
  invert1 : xbsIndex_r4/Inverter  en=off  latency=0  dbl_ovrd=off  block_type=inv
  invert2 : xbsIndex_r4/Inverter  en=off  latency=0  dbl_ovrd=off  block_type=inv
  invert3 : xbsIndex_r4/Inverter  en=off  latency=0  dbl_ovrd=off  block_type=inv
  slice1 : xbsIndex_r4/Slice  nbits=1  boolean_output=on  mode=Upper Bit Location + Width  bit1=0  base1=MSB of Input  bit0=0  base0=LSB of Input  dbl_ovrd=off  block_type=slice
  slice2 : xbsIndex_r4/Slice  nbits=1  boolean_output=on  mode=Upper Bit Location + Width  bit1=-1  base1=MSB of Input  bit0=0  base0=LSB of Input  dbl_ovrd=off  block_type=slice
  slice3 : xbsIndex_r4/Slice  nbits=1  boolean_output=on  mode=Upper Bit Location + Width  bit1=-2  base1=MSB of Input  bit0=0  base0=LSB of Input  dbl_ovrd=off  block_type=slice
  dout : Outport
  of : Outport  Port=2
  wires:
  din/1 -> convert/1(in), slice1/1, slice2/1, slice3/1
  convert/1(out) -> dout/1
  slice1/1 -> all_1s/1, invert1/1
  invert1/1 -> all_0s/1
  slice2/1 -> all_1s/2, invert2/1
  invert2/1 -> all_0s/2
  slice3/1 -> all_1s/3, invert3/1
  invert3/1 -> all_0s/3
  all_0s/1 -> and/1
  all_1s/1 -> and/2
  and/1 -> of/1

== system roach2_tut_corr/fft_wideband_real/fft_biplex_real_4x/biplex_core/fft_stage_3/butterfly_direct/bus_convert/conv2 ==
  din : Inport
  all_0s : xbsIndex_r4/Logical  logical_function=NAND  inputs=3  en=off  latency=1  precision=Full  arith_type=Unsigned  n_bits=16  bin_pt=0  align_bp=on  dbl_ovrd=off  block_type=logical
  all_1s : xbsIndex_r4/Logical  logical_function=NAND  inputs=3  en=off  latency=1  precision=Full  arith_type=Unsigned  n_bits=16  bin_pt=0  align_bp=on  dbl_ovrd=off  block_type=logical
  and : xbsIndex_r4/Logical  logical_function=AND  inputs=2  en=off  latency=0  precision=Full  arith_type=Unsigned  n_bits=16  bin_pt=0  align_bp=on  dbl_ovrd=off  block_type=logical
  convert : Subsystem  AncestorBlock=casper_library_misc/convert
  invert1 : xbsIndex_r4/Inverter  en=off  latency=0  dbl_ovrd=off  block_type=inv
  invert2 : xbsIndex_r4/Inverter  en=off  latency=0  dbl_ovrd=off  block_type=inv
  invert3 : xbsIndex_r4/Inverter  en=off  latency=0  dbl_ovrd=off  block_type=inv
  slice1 : xbsIndex_r4/Slice  nbits=1  boolean_output=on  mode=Upper Bit Location + Width  bit1=0  base1=MSB of Input  bit0=0  base0=LSB of Input  dbl_ovrd=off  block_type=slice
  slice2 : xbsIndex_r4/Slice  nbits=1  boolean_output=on  mode=Upper Bit Location + Width  bit1=-1  base1=MSB of Input  bit0=0  base0=LSB of Input  dbl_ovrd=off  block_type=slice
  slice3 : xbsIndex_r4/Slice  nbits=1  boolean_output=on  mode=Upper Bit Location + Width  bit1=-2  base1=MSB of Input  bit0=0  base0=LSB of Input  dbl_ovrd=off  block_type=slice
  dout : Outport
  of : Outport  Port=2
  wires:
  din/1 -> convert/1(in), slice1/1, slice2/1, slice3/1
  convert/1(out) -> dout/1
  slice1/1 -> all_1s/1, invert1/1
  invert1/1 -> all_0s/1
  slice2/1 -> all_1s/2, invert2/1
  invert2/1 -> all_0s/2
  slice3/1 -> all_1s/3, invert3/1
  invert3/1 -> all_0s/3
  all_0s/1 -> and/1
  all_1s/1 -> and/2
  and/1 -> of/1

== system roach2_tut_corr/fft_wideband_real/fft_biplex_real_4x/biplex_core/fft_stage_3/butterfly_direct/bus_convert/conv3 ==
  din : Inport
  all_0s : xbsIndex_r4/Logical  logical_function=NAND  inputs=3  en=off  latency=1  precision=Full  arith_type=Unsigned  n_bits=16  bin_pt=0  align_bp=on  dbl_ovrd=off  block_type=logical
  all_1s : xbsIndex_r4/Logical  logical_function=NAND  inputs=3  en=off  latency=1  precision=Full  arith_type=Unsigned  n_bits=16  bin_pt=0  align_bp=on  dbl_ovrd=off  block_type=logical
  and : xbsIndex_r4/Logical  logical_function=AND  inputs=2  en=off  latency=0  precision=Full  arith_type=Unsigned  n_bits=16  bin_pt=0  align_bp=on  dbl_ovrd=off  block_type=logical
  convert : Subsystem  AncestorBlock=casper_library_misc/convert
  invert1 : xbsIndex_r4/Inverter  en=off  latency=0  dbl_ovrd=off  block_type=inv
  invert2 : xbsIndex_r4/Inverter  en=off  latency=0  dbl_ovrd=off  block_type=inv
  invert3 : xbsIndex_r4/Inverter  en=off  latency=0  dbl_ovrd=off  block_type=inv
  slice1 : xbsIndex_r4/Slice  nbits=1  boolean_output=on  mode=Upper Bit Location + Width  bit1=0  base1=MSB of Input  bit0=0  base0=LSB of Input  dbl_ovrd=off  block_type=slice
  slice2 : xbsIndex_r4/Slice  nbits=1  boolean_output=on  mode=Upper Bit Location + Width  bit1=-1  base1=MSB of Input  bit0=0  base0=LSB of Input  dbl_ovrd=off  block_type=slice
  slice3 : xbsIndex_r4/Slice  nbits=1  boolean_output=on  mode=Upper Bit Location + Width  bit1=-2  base1=MSB of Input  bit0=0  base0=LSB of Input  dbl_ovrd=off  block_type=slice
  dout : Outport
  of : Outport  Port=2
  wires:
  din/1 -> convert/1(in), slice1/1, slice2/1, slice3/1
  convert/1(out) -> dout/1
  slice1/1 -> all_1s/1, invert1/1
  invert1/1 -> all_0s/1
  slice2/1 -> all_1s/2, invert2/1
  invert2/1 -> all_0s/2
  slice3/1 -> all_1s/3, invert3/1
  invert3/1 -> all_0s/3
  all_0s/1 -> and/1
  all_1s/1 -> and/2
  and/1 -> of/1

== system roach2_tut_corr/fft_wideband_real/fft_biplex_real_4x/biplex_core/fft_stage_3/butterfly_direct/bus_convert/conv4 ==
  din : Inport
  all_0s : xbsIndex_r4/Logical  logical_function=NAND  inputs=3  en=off  latency=1  precision=Full  arith_type=Unsigned  n_bits=16  bin_pt=0  align_bp=on  dbl_ovrd=off  block_type=logical
  all_1s : xbsIndex_r4/Logical  logical_function=NAND  inputs=3  en=off  latency=1  precision=Full  arith_type=Unsigned  n_bits=16  bin_pt=0  align_bp=on  dbl_ovrd=off  block_type=logical
  and : xbsIndex_r4/Logical  logical_function=AND  inputs=2  en=off  latency=0  precision=Full  arith_type=Unsigned  n_bits=16  bin_pt=0  align_bp=on  dbl_ovrd=off  block_type=logical
  convert : Subsystem  AncestorBlock=casper_library_misc/convert
  invert1 : xbsIndex_r4/Inverter  en=off  latency=0  dbl_ovrd=off  block_type=inv
  invert2 : xbsIndex_r4/Inverter  en=off  latency=0  dbl_ovrd=off  block_type=inv
  invert3 : xbsIndex_r4/Inverter  en=off  latency=0  dbl_ovrd=off  block_type=inv
  slice1 : xbsIndex_r4/Slice  nbits=1  boolean_output=on  mode=Upper Bit Location + Width  bit1=0  base1=MSB of Input  bit0=0  base0=LSB of Input  dbl_ovrd=off  block_type=slice
  slice2 : xbsIndex_r4/Slice  nbits=1  boolean_output=on  mode=Upper Bit Location + Width  bit1=-1  base1=MSB of Input  bit0=0  base0=LSB of Input  dbl_ovrd=off  block_type=slice
  slice3 : xbsIndex_r4/Slice  nbits=1  boolean_output=on  mode=Upper Bit Location + Width  bit1=-2  base1=MSB of Input  bit0=0  base0=LSB of Input  dbl_ovrd=off  block_type=slice
  dout : Outport
  of : Outport  Port=2
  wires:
  din/1 -> convert/1(in), slice1/1, slice2/1, slice3/1
  convert/1(out) -> dout/1
  slice1/1 -> all_1s/1, invert1/1
  invert1/1 -> all_0s/1
  slice2/1 -> all_1s/2, invert2/1
  invert2/1 -> all_0s/2
  slice3/1 -> all_1s/3, invert3/1
  invert3/1 -> all_0s/3
  all_0s/1 -> and/1
  all_1s/1 -> and/2
  and/1 -> of/1

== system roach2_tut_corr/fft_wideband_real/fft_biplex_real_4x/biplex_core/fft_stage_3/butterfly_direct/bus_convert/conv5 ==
  din : Inport
  all_0s : xbsIndex_r4/Logical  logical_function=NAND  inputs=3  en=off  latency=1  precision=Full  arith_type=Unsigned  n_bits=16  bin_pt=0  align_bp=on  dbl_ovrd=off  block_type=logical
  all_1s : xbsIndex_r4/Logical  logical_function=NAND  inputs=3  en=off  latency=1  precision=Full  arith_type=Unsigned  n_bits=16  bin_pt=0  align_bp=on  dbl_ovrd=off  block_type=logical
  and : xbsIndex_r4/Logical  logical_function=AND  inputs=2  en=off  latency=0  precision=Full  arith_type=Unsigned  n_bits=16  bin_pt=0  align_bp=on  dbl_ovrd=off  block_type=logical
  convert : Subsystem  AncestorBlock=casper_library_misc/convert
  invert1 : xbsIndex_r4/Inverter  en=off  latency=0  dbl_ovrd=off  block_type=inv
  invert2 : xbsIndex_r4/Inverter  en=off  latency=0  dbl_ovrd=off  block_type=inv
  invert3 : xbsIndex_r4/Inverter  en=off  latency=0  dbl_ovrd=off  block_type=inv
  slice1 : xbsIndex_r4/Slice  nbits=1  boolean_output=on  mode=Upper Bit Location + Width  bit1=0  base1=MSB of Input  bit0=0  base0=LSB of Input  dbl_ovrd=off  block_type=slice
  slice2 : xbsIndex_r4/Slice  nbits=1  boolean_output=on  mode=Upper Bit Location + Width  bit1=-1  base1=MSB of Input  bit0=0  base0=LSB of Input  dbl_ovrd=off  block_type=slice
  slice3 : xbsIndex_r4/Slice  nbits=1  boolean_output=on  mode=Upper Bit Location + Width  bit1=-2  base1=MSB of Input  bit0=0  base0=LSB of Input  dbl_ovrd=off  block_type=slice
  dout : Outport
  of : Outport  Port=2
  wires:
  din/1 -> convert/1(in), slice1/1, slice2/1, slice3/1
  convert/1(out) -> dout/1
  slice1/1 -> all_1s/1, invert1/1
  invert1/1 -> all_0s/1
  slice2/1 -> all_1s/2, invert2/1
  invert2/1 -> all_0s/2
  slice3/1 -> all_1s/3, invert3/1
  invert3/1 -> all_0s/3
  all_0s/1 -> and/1
  all_1s/1 -> and/2
  and/1 -> of/1

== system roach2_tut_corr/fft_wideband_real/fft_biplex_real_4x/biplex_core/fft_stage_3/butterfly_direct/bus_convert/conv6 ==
  din : Inport
  all_0s : xbsIndex_r4/Logical  logical_function=NAND  inputs=3  en=off  latency=1  precision=Full  arith_type=Unsigned  n_bits=16  bin_pt=0  align_bp=on  dbl_ovrd=off  block_type=logical
  all_1s : xbsIndex_r4/Logical  logical_function=NAND  inputs=3  en=off  latency=1  precision=Full  arith_type=Unsigned  n_bits=16  bin_pt=0  align_bp=on  dbl_ovrd=off  block_type=logical
  and : xbsIndex_r4/Logical  logical_function=AND  inputs=2  en=off  latency=0  precision=Full  arith_type=Unsigned  n_bits=16  bin_pt=0  align_bp=on  dbl_ovrd=off  block_type=logical
  convert : Subsystem  AncestorBlock=casper_library_misc/convert
  invert1 : xbsIndex_r4/Inverter  en=off  latency=0  dbl_ovrd=off  block_type=inv
  invert2 : xbsIndex_r4/Inverter  en=off  latency=0  dbl_ovrd=off  block_type=inv
  invert3 : xbsIndex_r4/Inverter  en=off  latency=0  dbl_ovrd=off  block_type=inv
  slice1 : xbsIndex_r4/Slice  nbits=1  boolean_output=on  mode=Upper Bit Location + Width  bit1=0  base1=MSB of Input  bit0=0  base0=LSB of Input  dbl_ovrd=off  block_type=slice
  slice2 : xbsIndex_r4/Slice  nbits=1  boolean_output=on  mode=Upper Bit Location + Width  bit1=-1  base1=MSB of Input  bit0=0  base0=LSB of Input  dbl_ovrd=off  block_type=slice
  slice3 : xbsIndex_r4/Slice  nbits=1  boolean_output=on  mode=Upper Bit Location + Width  bit1=-2  base1=MSB of Input  bit0=0  base0=LSB of Input  dbl_ovrd=off  block_type=slice
  dout : Outport
  of : Outport  Port=2
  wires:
  din/1 -> convert/1(in), slice1/1, slice2/1, slice3/1
  convert/1(out) -> dout/1
  slice1/1 -> all_1s/1, invert1/1
  invert1/1 -> all_0s/1
  slice2/1 -> all_1s/2, invert2/1
  invert2/1 -> all_0s/2
  slice3/1 -> all_1s/3, invert3/1
  invert3/1 -> all_0s/3
  all_0s/1 -> and/1
  all_1s/1 -> and/2
  and/1 -> of/1

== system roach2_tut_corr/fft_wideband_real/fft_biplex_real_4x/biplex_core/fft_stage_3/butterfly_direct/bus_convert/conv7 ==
  din : Inport
  all_0s : xbsIndex_r4/Logical  logical_function=NAND  inputs=3  en=off  latency=1  precision=Full  arith_type=Unsigned  n_bits=16  bin_pt=0  align_bp=on  dbl_ovrd=off  block_type=logical
  all_1s : xbsIndex_r4/Logical  logical_function=NAND  inputs=3  en=off  latency=1  precision=Full  arith_type=Unsigned  n_bits=16  bin_pt=0  align_bp=on  dbl_ovrd=off  block_type=logical
  and : xbsIndex_r4/Logical  logical_function=AND  inputs=2  en=off  latency=0  precision=Full  arith_type=Unsigned  n_bits=16  bin_pt=0  align_bp=on  dbl_ovrd=off  block_type=logical
  convert : Subsystem  AncestorBlock=casper_library_misc/convert
  invert1 : xbsIndex_r4/Inverter  en=off  latency=0  dbl_ovrd=off  block_type=inv
  invert2 : xbsIndex_r4/Inverter  en=off  latency=0  dbl_ovrd=off  block_type=inv
  invert3 : xbsIndex_r4/Inverter  en=off  latency=0  dbl_ovrd=off  block_type=inv
  slice1 : xbsIndex_r4/Slice  nbits=1  boolean_output=on  mode=Upper Bit Location + Width  bit1=0  base1=MSB of Input  bit0=0  base0=LSB of Input  dbl_ovrd=off  block_type=slice
  slice2 : xbsIndex_r4/Slice  nbits=1  boolean_output=on  mode=Upper Bit Location + Width  bit1=-1  base1=MSB of Input  bit0=0  base0=LSB of Input  dbl_ovrd=off  block_type=slice
  slice3 : xbsIndex_r4/Slice  nbits=1  boolean_output=on  mode=Upper Bit Location + Width  bit1=-2  base1=MSB of Input  bit0=0  base0=LSB of Input  dbl_ovrd=off  block_type=slice
  dout : Outport
  of : Outport  Port=2
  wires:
  din/1 -> convert/1(in), slice1/1, slice2/1, slice3/1
  convert/1(out) -> dout/1
  slice1/1 -> all_1s/1, invert1/1
  invert1/1 -> all_0s/1
  slice2/1 -> all_1s/2, invert2/1
  invert2/1 -> all_0s/2
  slice3/1 -> all_1s/3, invert3/1
  invert3/1 -> all_0s/3
  all_0s/1 -> and/1
  all_1s/1 -> and/2
  and/1 -> of/1

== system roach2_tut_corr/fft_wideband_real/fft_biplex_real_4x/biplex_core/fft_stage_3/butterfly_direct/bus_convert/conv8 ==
  din : Inport
  all_0s : xbsIndex_r4/Logical  logical_function=NAND  inputs=3  en=off  latency=1  precision=Full  arith_type=Unsigned  n_bits=16  bin_pt=0  align_bp=on  dbl_ovrd=off  block_type=logical
  all_1s : xbsIndex_r4/Logical  logical_function=NAND  inputs=3  en=off  latency=1  precision=Full  arith_type=Unsigned  n_bits=16  bin_pt=0  align_bp=on  dbl_ovrd=off  block_type=logical
  and : xbsIndex_r4/Logical  logical_function=AND  inputs=2  en=off  latency=0  precision=Full  arith_type=Unsigned  n_bits=16  bin_pt=0  align_bp=on  dbl_ovrd=off  block_type=logical
  convert : Subsystem  AncestorBlock=casper_library_misc/convert
  invert1 : xbsIndex_r4/Inverter  en=off  latency=0  dbl_ovrd=off  block_type=inv
  invert2 : xbsIndex_r4/Inverter  en=off  latency=0  dbl_ovrd=off  block_type=inv
  invert3 : xbsIndex_r4/Inverter  en=off  latency=0  dbl_ovrd=off  block_type=inv
  slice1 : xbsIndex_r4/Slice  nbits=1  boolean_output=on  mode=Upper Bit Location + Width  bit1=0  base1=MSB of Input  bit0=0  base0=LSB of Input  dbl_ovrd=off  block_type=slice
  slice2 : xbsIndex_r4/Slice  nbits=1  boolean_output=on  mode=Upper Bit Location + Width  bit1=-1  base1=MSB of Input  bit0=0  base0=LSB of Input  dbl_ovrd=off  block_type=slice
  slice3 : xbsIndex_r4/Slice  nbits=1  boolean_output=on  mode=Upper Bit Location + Width  bit1=-2  base1=MSB of Input  bit0=0  base0=LSB of Input  dbl_ovrd=off  block_type=slice
  dout : Outport
  of : Outport  Port=2
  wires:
  din/1 -> convert/1(in), slice1/1, slice2/1, slice3/1
  convert/1(out) -> dout/1
  slice1/1 -> all_1s/1, invert1/1
  invert1/1 -> all_0s/1
  slice2/1 -> all_1s/2, invert2/1
  invert2/1 -> all_0s/2
  slice3/1 -> all_1s/3, invert3/1
  invert3/1 -> all_0s/3
  all_0s/1 -> and/1
  all_1s/1 -> and/2
  and/1 -> of/1
